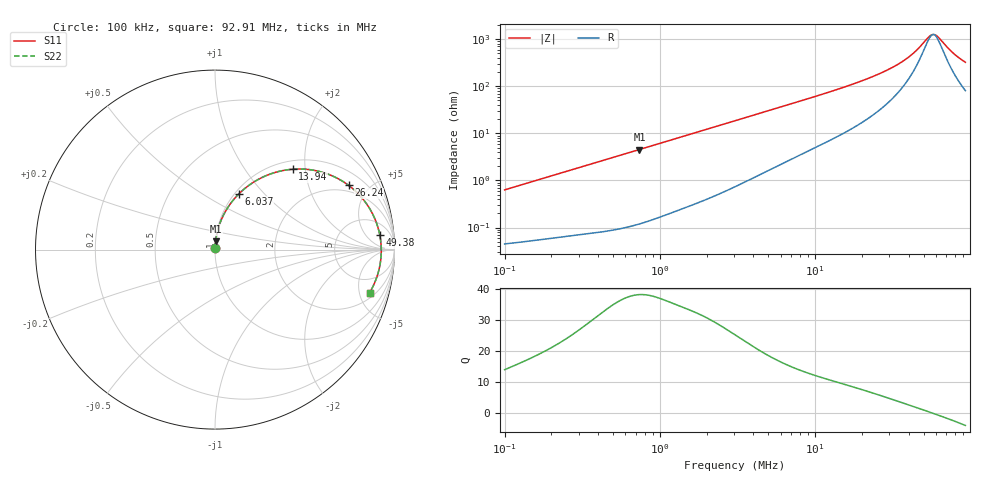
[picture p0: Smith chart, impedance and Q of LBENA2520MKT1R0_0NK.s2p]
! LBENA2520MKT1R0_0NK  S-PARAMETER MODEL  ( General Type )
! Model Generated by TAIYO YUDEN Corporation (http://www.ty-top.com)
! Version 1.0
! TAIYO YUDEN Control No. 211116
! Copyright(c) 2021 TAIYO YUDEN CO.,LTD. All Rights Reserved.
! Product Description (link to TY-COMPAS)
! https://ds.yuden.co.jp/TYCOMPAS/or/detail?pn=LBENA2520MKT1R0M0NK&u=M
! Products Name : Inductors
! Characteristics :
!  Inductance : 1.0 uH , SRF(min) : -Hz , DC Resistance(max) : 0.042 Ohm
!  Rated Current : Saturation :4400 mA , Temp Rise : 3200 mA
!  Case Size : 2.5 x 2.0 / 0.098 x 0.079 [mm/inch] , Thickness : 1.2 / 0.047 [mm/inch]
!  (Conditions: Temperature = 25 degC , DC Bias Current/Voltage = 0A / 0V)
! External Node Assignments :
!  1  o---GGG---o  2
! GND o---------o GND
! Frequency Range : 0.1MHz  -  92.907885MHz  [ 402 STEP ]
# MHz S RI R 50
! Freq[MHz].  S11 Real  S11 Imag  S21 Real  S21 Imag  S12 Real  S12 Imag  S22 Real  S22 Imag
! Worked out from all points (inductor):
!   401 points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, 100 kHz to 92.91 MHz, reference 50 ohm
!   read as one part in series: L = 998 nH near 103.5 kHz
!   highest Q = 38.1 at 738.2 kHz (marker M1), where L = 978 nH
!   self-resonance near 57.71 MHz
!   S11 on the Smith chart (normalised r, x): 100 kHz: 1.00, +0.01; 6.037 MHz: 1.04, +0.73; 13.94 MHz: 1.17, +1.71; 26.24 MHz: 1.64, +3.70; 49.38 MHz: 11, +12; 92.91 MHz: 2.62, -6.26
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0.1  0.000488 0.00629  0.9995 -0.00629  0.9995 -0.00629  0.000488 0.00629
0.314158  0.00108 0.0194  0.9989 -0.0194  0.9989 -0.0194  0.00108 0.0194
0.738168  0.00324 0.0452  0.9968 -0.0452  0.9968 -0.0452  0.00324 0.0452
0.986956  0.00527 0.0601  0.9947 -0.0601  0.9947 -0.0601  0.00527 0.0601
1.82567  0.0156 0.1092  0.9844 -0.1092  0.9844 -0.1092  0.0156 0.1092
3.100605  0.041 0.1792  0.959 -0.1792  0.959 -0.1792  0.041 0.1792
6.037144  0.132 0.3094  0.868 -0.3094  0.868 -0.3094  0.132 0.3094
9.575801  0.2679 0.4046  0.7321 -0.4046  0.7321 -0.4046  0.2679 0.4046
13.94498  0.4324 0.4478  0.5676 -0.4478  0.5676 -0.4478  0.4324 0.4478
19.29303  0.5973 0.4311  0.4027 -0.4311  0.4027 -0.4311  0.5973 0.4311
26.23994  0.7445 0.3581  0.2555 -0.3581  0.2555 -0.3581  0.7445 0.3581
30.08319  0.7997 0.3094  0.2003 -0.3094  0.2003 -0.3094  0.7997 0.3094
35.08367  0.8511 0.2455  0.1489 -0.2455  0.1489 -0.2455  0.8511 0.2455
39.54085  0.8822 0.1905  0.1178 -0.1905  0.1178 -0.1905  0.8822 0.1905
44.56428  0.9053 0.1322  0.0947 -0.1322  0.0947 -0.1322  0.9053 0.1322
49.37507  0.9184 0.0805  0.0816 -0.0805  0.0816 -0.0805  0.9184 0.0805
55.64788  0.9259 0.0189  0.0741 -0.0189  0.0741 -0.0189  0.9259 0.0189
59.58393  0.9263 -0.0166  0.0737 0.0166  0.0737 0.0166  0.9263 -0.0166
62.71762  0.9249 -0.0432  0.0751 0.0432  0.0751 0.0432  0.9249 -0.0432
76.98943  0.9034 -0.1483  0.0966 0.1483  0.0966 0.1483  0.9034 -0.1483
85.30057  0.8832 -0.199  0.1168 0.199  0.1168 0.199  0.8832 -0.199
92.90788  0.8616 -0.2396  0.1384 0.2396  0.1384 0.2396  0.8616 -0.2396
